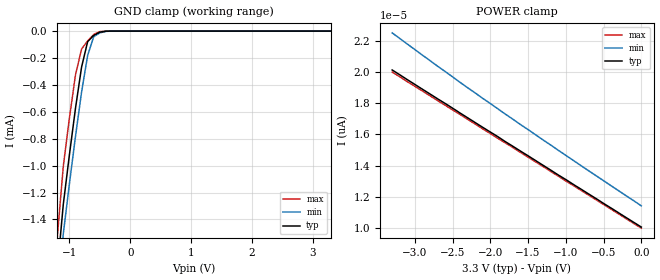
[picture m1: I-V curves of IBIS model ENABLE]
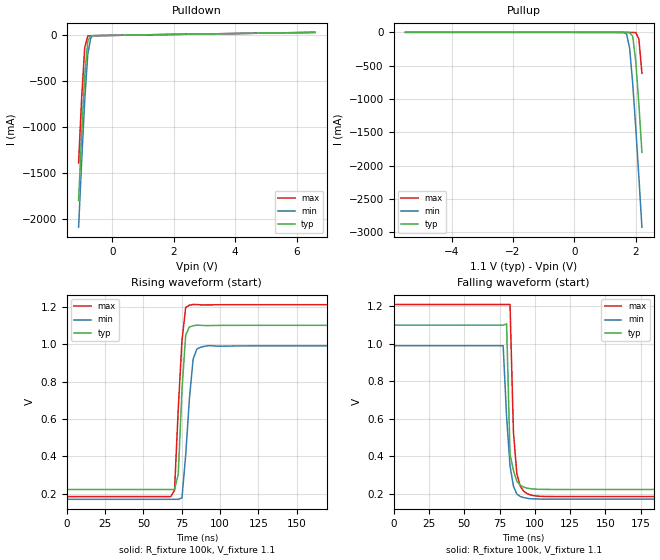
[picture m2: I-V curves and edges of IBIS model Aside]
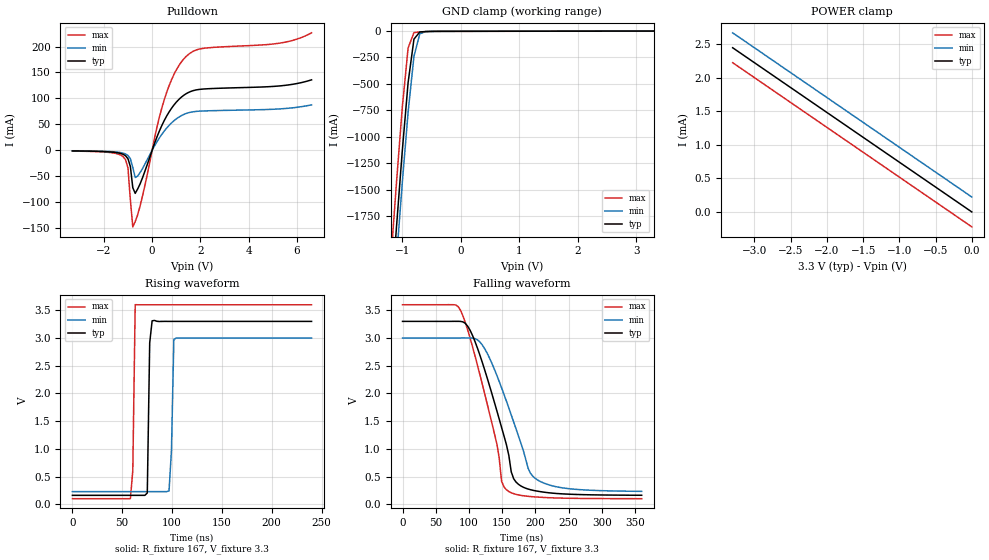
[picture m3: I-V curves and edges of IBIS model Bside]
| PCA9519 - IBIS model
| Note on Port A behavior:
| Since port A (low voltage side) has an internal pull up current source and a
| 200 ohm pull down driver as documented in the datasheet, the pull down curve
| will have a nearly linear behavior since the pull down is dominated by the
| 200ohm resistive path.
[IBIS Ver]   4.0
[Comment Char]   |_char
| Aside = 1.1V Bside = 3.3V
[File name]   pca9519_a1_1b_3_3.ibs
[File Rev]   1
[Date]   Sept 23, 2009 3:25:44 PM
[Source]
[Notes]
|The package model information is simulated at 400 kHz,
|which is the maximum system operating frequency.
[Disclaimer]
(C) Copyright 2007 NXP Semiconductors
All rights reserved
NXP Semiconductors (NXP) does not warrant that this model and any other
accompanying information (Model) accurately or fully represents the
operating characteristics and specifications of the semiconductor
products to which the Model relates.  Moreover, the Model is furnished
on an "as is" and with "all faults" basis, and without support or
warranty of any kind.  NXP disclaims all warranties, whether expressed
or implied or statutory, including without limitation all implied
warranties of non-infringement, merchantability and fitness for any
purpose, and those arising from a course of dealing or usage of trade.
NXP does not convey any license under its or any third party's patents,
copyrights or other intellectual property or proprietary rights.
You and your company assume any and all risks and liability arising out
of the application or use of the Model.
In no event shall NXP be liable for any direct, indirect, special,
consequential or incidental damages, however caused, whether in
warranty, contract or tort (including negligence), strict liability or
other legal theory, including, without limitation, for lost profits,
business interruption, or corruption or loss of data or information,
arising out of or in connection with the use of or the inability to use
the Model, even if NXP has been advised of the possibility of such
damages.
NXP provides the Model as a courtesy to our customers. You and your
company shall not distribute, convey, sell, or give the Model to anyone
else without receiving prior written permission from NXP.
NXP reserves the right to make changes without notice to the Model to
improve reliability, function, or design.
Please be aware that your receipt and subsequent use of the Model shall
serve as acceptance of these terms and conditions.  If you do not
accept these terms, return or destroy the Model immediately.
[Copyright]
(C) Copyright 2009 NXP Semiconductors  All rights reserved
| HVQFN24 - package
[Component]   PCA9519BS
Si_location Die
Timing_location Pin
[Manufacturer]   NXP Semiconductors
[Package]
|variable   typ   min   max
R_pkg   3.74E-03   3.16E-03   4.32E-03
L_pkg   1.22E-09   0.99E-09   1.45E-09
C_pkg   0.20E-12   0.18E-12   0.22E-12
[Pin] signal_name   model_name   R_pin   L_pin   C_pin
1   A2   Aside   4.32E-03  1.45E-09  0.22E-12
2   A3   Aside   3.88E-03  1.27E-09  0.21E-12
3   A4   Aside   3.68E-03  1.18E-09  0.20E-12
4   A5   Aside   3.68E-03  1.18E-09  0.20E-12
5   A6   Aside   3.88E-03  1.26E-09  0.21E-12
6   A7   Aside   4.30E-03  1.44E-09  0.22E-12
7   A8   Aside   4.15E-03  1.40E-09  0.21E-12
8   NC   NC   NA   NA   NA
9   NC   NC   NA   NA   NA
10   VCCB   POWER   3.16E-03  0.99E-09  0.18E-12
11   EN   ENABLE   3.31E-03  1.06E-09  0.19E-12
12   B8   Bside   4.15E-03  1.39E-09  0.22E-12
13   B7   Bside   4.33E-03  1.45E-09  0.22E-12
14   B6   Bside   3.90E-03  1.27E-09  0.21E-12
15   B5   Bside   3.69E-03  1.18E-09  0.20E-12
16   B4   Bside   3.68E-03  1.18E-09  0.20E-12
17   B3   Bside   3.88E-03  1.26E-09  0.21E-12
18   B2   Bside   4.29E-03  1.44E-09  0.22E-12
19   B1   Bside   4.12E-03  1.39E-09  0.21E-12
20   NC   NC   NA   NA   NA
21   NC   NC   NA   NA   NA
22   GND   GND   3.20E-03  1.01E-09  0.18E-12
23   VCCA   POWER   3.37E-03  1.08E-09  0.19E-12
24   A1   Aside   4.12E-03  1.38E-09  0.21E-12
[Package Model]   hvqfn24_sot616ac2
|The package model information is simulated at 400 kHz,
|which is the maximum system operating frequency.
| TSSOP8 - package
[Component]   PCA9519PW
Si_location Die
Timing_location Pin
[Manufacturer]   NXP Semiconductors
[Package]
|variable   typ   min   max
R_pkg   4.66E-03   4.03E-03   5.28E-03
L_pkg   2.39E-09   1.87E-09   2.90E-09
C_pkg   0.36E-12   0.30E-12   0.42E-12
[Pin] signal_name   model_name   R_pin   L_pin   C_pin
1   EN   ENABLE   4.30E-03  2.79E-09  0.42E-12
2   B1   Bside   4.95E-03  2.58E-09  0.41E-12
3   B2   Bside   5.28E-03  2.39E-09  0.35E-12
4   B3   Bside   4.59E-03  2.08E-09  0.32E-12
5   B4   Bside   4.04E-03  1.87E-09  0.30E-12
6   B5   Bside   4.03E-03  1.87E-09  0.30E-12
7   B6   Bside   4.57E-03  2.07E-09  0.32E-12
8   B7   Bside   5.26E-03  2.38E-09  0.35E-12
9   B8   Bside   4.87E-03  2.56E-09  0.41E-12
10   GND   GND   4.39E-03  2.85E-09  0.42E-12
11   VCCA   POWER   4.33E-03  2.81E-09  0.42E-12
12   A8   Aside   4.88E-03  2.56E-09  0.41E-12
13   A7   Aside   5.28E-03  2.38E-09  0.35E-12
14   A6   Aside   4.56E-03  2.07E-09  0.32E-12
15   A5   Aside   4.03E-03  1.87E-09  0.30E-12
16   A4   Aside   4.04E-03  1.88E-09  0.30E-12
17   A3   Aside   4.58E-03  2.09E-09  0.32E-12
18   A2   Aside   5.28E-03  2.39E-09  0.35E-12
19   A1   Aside   4.91E-03  2.57E-09  0.41E-12
20   VCCB   POWER   4.46E-03  2.90E-09  0.42E-12
[Package Model]   tssop20_sot360db7
|   PACKAGE MODEL HVQFN24
[Define Package Model]   hvqfn24_sot616ac2
[Manufacturer]  NXP
[OEM]  NXP
[Description]   Full package IBIS model.Simulated @ 400kHz
[Number Of Pins]  20
[Pin Numbers]
|Pin Num   Terminal Name
1   | Lead1:pin1
2   | Lead2:pin2
3   | Lead3:pin3
4   | Lead4:pin4
5   | Lead5:pin5
6   | Lead6:pin6
7   | Lead7:pin7
8   | Lead10:pin8
9   | Lead11:pin9
10   | Lead12:pin10
11   | Lead13:pin11
12   | Lead14:pin12
13   | Lead15:pin13
14   | Lead16:pin14
15   | Lead17:pin15
16   | Lead18:pin16
17   | Lead19:pin17
18   | Lead22:pin18
19   | Lead23:pin19
20   | Lead24:pin20
[Model Data]
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[End Model Data]
[End Package Model]
|   PACKAGE MODEL TSSOP20
[Define Package Model]  tssop20_sot360db7
[Manufacturer]  NXP
[OEM] NXP
[Description]   Full package IBIS model.Simulated @ 400kHz
[Number Of Pins]  20
[Pin Numbers]
|Pin Num   Terminal Name
1   | Lead1:pin1
2   | Lead2:pin2
3   | Lead3:pin3
4   | Lead4:pin4
5   | Lead5:pin5
6   | Lead6:pin6
7   | Lead7:pin7
8   | Lead8:pin8
9   | Lead9:pin9
10   | Lead10:pin10
11   | Lead11:pin11
12   | Lead12:pin12
13   | Lead13:pin13
14   | Lead14:pin14
15   | Lead15:pin15
16   | Lead16:pin16
17   | Lead17:pin17
18   | Lead18:pin18
19   | Lead19:pin19
20   | Lead20:pin20
[Model Data]
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[End Model Data]
[End Package Model]
| Models and submodels in the file (3): ENABLE (Input), Aside (I/O), Bside (I/O_open_drain)
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|The package model information is simulated at 400 kHz,
|which is the maximum system operating frequency.
[Model]   ENABLE
Model_type Input
Vinh=2.1
Vinl=0.9
|variable   typ   min   max
C_comp   1.84p   1.81p   1.86p
[Temperature Range] 27   85   -40
[Voltage Range]   3.3   3   3.6
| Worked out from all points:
|   GND clamp passes 1 mA (typ) near -1.02 V on its own axis
[GND Clamp]
-3.3V     -14.99A    -14.5A     -15.58A
-1.2V     -1.787mA   -1.999mA   -1.54mA
-1.1V     -1.288mA   -1.507mA   -1.005mA
-1V       -921.3uA   -1.137mA   -647uA
-900mV    -574.4uA   -783.6uA   -327uA
-800mV    -268uA     -454.2uA   -133.1uA
-700mV    -78.19uA   -180.8uA   -72.93uA
-600mV    -31.83uA   -40.83uA   -25.26uA
-500mV    -8.452uA   -13.3uA    -3.68uA
-400mV    -758.4nA   -2.213uA   -96.83nA
-300mV    -18.6nA    -106.4nA   -805.3pA
3.3V      10.06pA    11.42pA    9.99pA
[POWER Clamp]
-3.3V     20.12pA    22.49pA    19.98pA
-2.4V     17.36pA    19.32pA    17.27pA
-1.8V     15.53pA    17.29pA    15.44pA
0V        10.06pA    11.42pA    9.99pA
[Model]   Aside
Model_type I/O
Enable Active-High
Vinh=0.7
Vinl=0.2
Vref=1.1
Vmeas=0.55
Rref=100k
Cref=20p
|variable   typ   min   max
C_comp   8.4p   8.2p   8.6p
[Model Spec]
Vinh   0.77   0.7   1.21
Vinl   0.15   0.15   0.3
[Temperature Range] 27   85   -40
[Voltage Range]   1.1   0.99   1.21
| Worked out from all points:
|   slope of the pulldown table from 0 to 0.165 V, typ, clamps not added: 204 ohm
|   slope of the pullup table from 0 to 0.165 V, typ, clamps not added: 296 ohm
|   falling waveform, R_fixture 100k, V_fixture 1.1: 20-80 % time 2.17ns typ, 4.12ns min, 3.2ns max; typ from 1.1 V to 0.224 V
|   rising waveform, R_fixture 100k, V_fixture 1.1: 20-80 % time 3.33ns typ, 4.54ns min, 3.8ns max; typ from 0.223 V to 1.1 V
[Pullup]
-5.5V     66.77uA    65.4uA     71.68uA
1.5V      -1.142mA   -1.212mA   -931.2uA
1.6V      -1.323mA   -2.757mA   -940.8uA
1.7V      -1.665mA   -25.03mA   -1.032mA
1.8V      -3.985mA   -238.2mA   -1.3mA
1.9V      -58.74mA   -766.2mA   -1.665mA
2V        -438.6mA   -1.437A    -3.737mA
2.1V      -1.076A    -2.164A    -98.31mA
2.2V      -1.798A    -2.92A     -613.2mA
[Pulldown]
-1.1V     -1.798A    -2.09A     -1.391A
-1V       -1.076A    -1.367A    -679.7mA
-900mV    -439.5mA   -705.3mA   -132.4mA
-800mV    -60.85mA   -201.9mA   -7.514mA
-700mV    -6.497mA   -21.57mA   -4.406mA
-600mV    -4.062mA   -4.617mA   -3.889mA
-500mV    -3.529mA   -3.237mA   -3.393mA
6.6V      31.82mA    31.06mA    32.37mA
[Falling Waveform]
R_fixture=100k
V_fixture=1.1
V_fixture_min=0.99
V_fixture_max=1.21
0s        1.1V       990mV      1.21V
77.58ns   1.1V       990mV      1.21V
80ns      1.107V     612mV      1.21V
82.42ns   413.1mV    349.7mV    1.21V
84.85ns   325.2mV    241.5mV    530.1mV
87.27ns   267.9mV    199.6mV    306.8mV
89.7ns    247mV      186.6mV    240.9mV
94.55ns   231.1mV    177mV      201.6mV
109.1ns   224.4mV    172.7mV    186.6mV
240ns     224mV      171.5mV    186.2mV
[Rising Waveform]
R_fixture=100k
V_fixture=1.1
V_fixture_min=0.99
V_fixture_max=1.21
0s        223.5mV    171.4mV    185.8mV
67.88ns   223.5mV    171.4mV    185.8mV
70.3ns    223.2mV    171.4mV    219.8mV
72.73ns   305.6mV    171.2mV    651.9mV
75.15ns   754.9mV    178.9mV    1.019V
77.58ns   1.047V     405.6mV    1.195V
80ns      1.091V     706.8mV    1.207V
82.42ns   1.097V     919.4mV    1.211V
89.7ns    1.099V     987.8mV    1.209V
240ns     1.1V       990mV      1.21V
[Ramp]
R_load=100k
dV/dt_r   5.206E-1/2.934E-9   4.858E-1/4.060E-9   6.093E-1/3.782E-9
dV/dt_f   5.256E-1/2.702E-9   4.911E-1/3.093E-9   6.143E-1/2.049E-9
|[End   Aside
[Model]   Bside
Model_type I/O_open_drain
Enable Active-High
Vinh=2.1
Vinl=0.9
Vref=3.3
Vmeas=1.65
Rref=167
Cref=57p
|variable   typ   min   max
C_comp   7.72p   7.7p   7.74p
[Model Spec]
Vinh   2.31   2.1   3.6
Vinl   0.99   0.9   1.08
[Temperature Range] 27   85   -40
[Voltage Range]   3.3   3   3.6
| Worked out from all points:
|   slope of the pulldown table from 0 to 0.495 V, typ, clamps not added: 8.73 ohm
|   POWER clamp passes 1 mA (typ) near -1.35 V on its own axis
|   falling waveform, R_fixture 167, V_fixture 3.3: 20-80 % time 44.2ns typ, 48.1ns min, 41.8ns max; typ from 3.3 V to 0.164 V
|   rising waveform, R_fixture 167, V_fixture 3.3: 20-80 % time 1.69ns typ, 2.39ns min, 1.7ns max; typ from 0.162 V to 3.3 V
[Pulldown]
-3.3V     -1.114mA   -877uA     -1.459mA
-1.2V     -7.664mA   -5.367mA   -12.12mA
-1V       -16.14mA   -9.967mA   -33.64mA
-900mV    -31.19mA   -16.36mA   -95.85mA
-800mV    -72.05mA   -32.98mA   -147.4mA
-700mV    -82.88mA   -52.36mA   -137.3mA
-600mV    -74.54mA   -49.66mA   -124.4mA
500mV     57.17mA    37.02mA    97.16mA
1.3V      105.7mA    68.94mA    175.5mA
2V        117.6mA    75.59mA    195.6mA
5.2V      123.8mA    79.59mA    206mA
6.6V      135.8mA    87.62mA    226.4mA
[GND Clamp]
-3.3V     -19.69A    -19.93A    -19.34A
-1.2V     -2.622A    -2.922A    -2.204A
-1.1V     -1.862A    -2.165A    -1.442A
-1V       -1.136A    -1.438A    -725.8mA
-900mV    -487.5mA   -767.1mA   -159.6mA
-800mV    -76.17mA   -238.8mA   -14.56mA
-700mV    -8.529mA   -26.2mA    -8.505mA
-600mV    -4.951mA   -5.06mA    -4.826mA
3.3V      158.9pA    222.2uA    -222.2uA
[POWER Clamp]
-3.3V     2.444mA    2.667mA    2.222mA
-2V       1.481mA    1.704mA    1.259mA
-1.9V     1.407mA    1.63mA     1.185mA
0V        158.9pA    222.2uA    -222.2uA
[Falling Waveform]
R_fixture=167
V_fixture=3.3
V_fixture_min=3
V_fixture_max=3.6
0s        3.3V       3V         3.6V
87.27ns   3.299V     3V         3.5V
120ns     2.563V     2.876V     2.172V
141.8ns   1.695V     2.331V     1.101V
149.1ns   1.388V     2.102V     418.6mV
156.4ns   1.078V     1.862V     263.3mV
167.3ns   462.4mV    1.487V     192.6mV
189.1ns   275.7mV    647.9mV    144.4mV
203.6ns   236.4mV    436.6mV    130.6mV
360ns     163.8mV    234.1mV    102mV
[Rising Waveform]
R_fixture=167
V_fixture=3.3
V_fixture_min=3
V_fixture_max=3.6
0s        161.6mV    228.3mV    101.2mV
58.18ns   161.6mV    228.3mV    101.2mV
60.61ns   161.6mV    228.3mV    605.9mV
63.03ns   161.6mV    228.3mV    3.602V
75.15ns   203.9mV    228.3mV    3.6V
77.58ns   2.912V     228.3mV    3.6V
80ns      3.31V      228.3mV    3.6V
96.97ns   3.3V       240.5mV    3.6V
101.8ns   3.3V       2.975V     3.6V
240ns     3.3V       3V         3.6V
[Ramp]
R_load=1350
dV/dt_r   1.959E+0/1.367E-9   1.770E+0/1.646E-9   2.147E+0/1.168E-9
dV/dt_f   1.959E+0/2.998E-8   1.769E+0/2.975E-8   2.147E+0/3.149E-8
|[End   Bside
